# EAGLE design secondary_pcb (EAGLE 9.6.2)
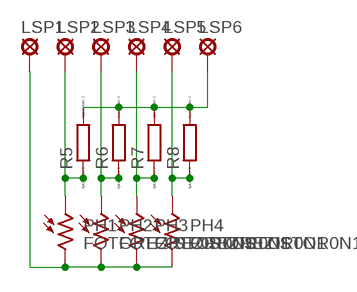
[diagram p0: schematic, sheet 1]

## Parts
LSP1  SVORKA_2,3/0,8  [LSP10]
LSP2  SVORKA_2,3/0,8  [LSP10]
LSP3  SVORKA_2,3/0,8  [LSP10]
LSP4  SVORKA_2,3/0,8  [LSP10]
LSP5  SVORKA_2,3/0,8  [LSP10]
LSP6  SVORKA_2,3/0,8  [LSP10]
PH1  FOTOREZISTOR0N1  [VT800]
PH2  FOTOREZISTOR0N1  [VT800]
PH3  FOTOREZISTOR0N1  [VT800]
PH4  FOTOREZISTOR0N1  [VT800]
R5  R0207/10  [0207/10]
R6  R0207/10  [0207/10]
R7  R0207/10  [0207/10]
R8  R0207/10  [0207/10]

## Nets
N$1: LSP1.MP PH1.2 PH2.2 PH3.2 PH4.2
N$2: LSP2.MP PH1.1 R5.1
N$3: LSP3.MP PH2.1 R6.1
N$4: LSP4.MP PH3.1 R7.1
N$5: LSP5.MP PH4.1 R8.1
N$6: LSP6.MP R5.2 R6.2 R7.2 R8.2

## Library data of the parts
LSP1-LSP6 = knihovna praxe 123:SVORKA_2,3/0,8: SOLDER PAD
PH1-PH4 = knihovna praxe 123:FOTOREZISTOR: Photoconductive Cell VT800 Series
R5-R8 = eagle-ltspice:R: RESISTOR, European symbol; SPICEMODEL: NONE; SPICEPREFIX: R

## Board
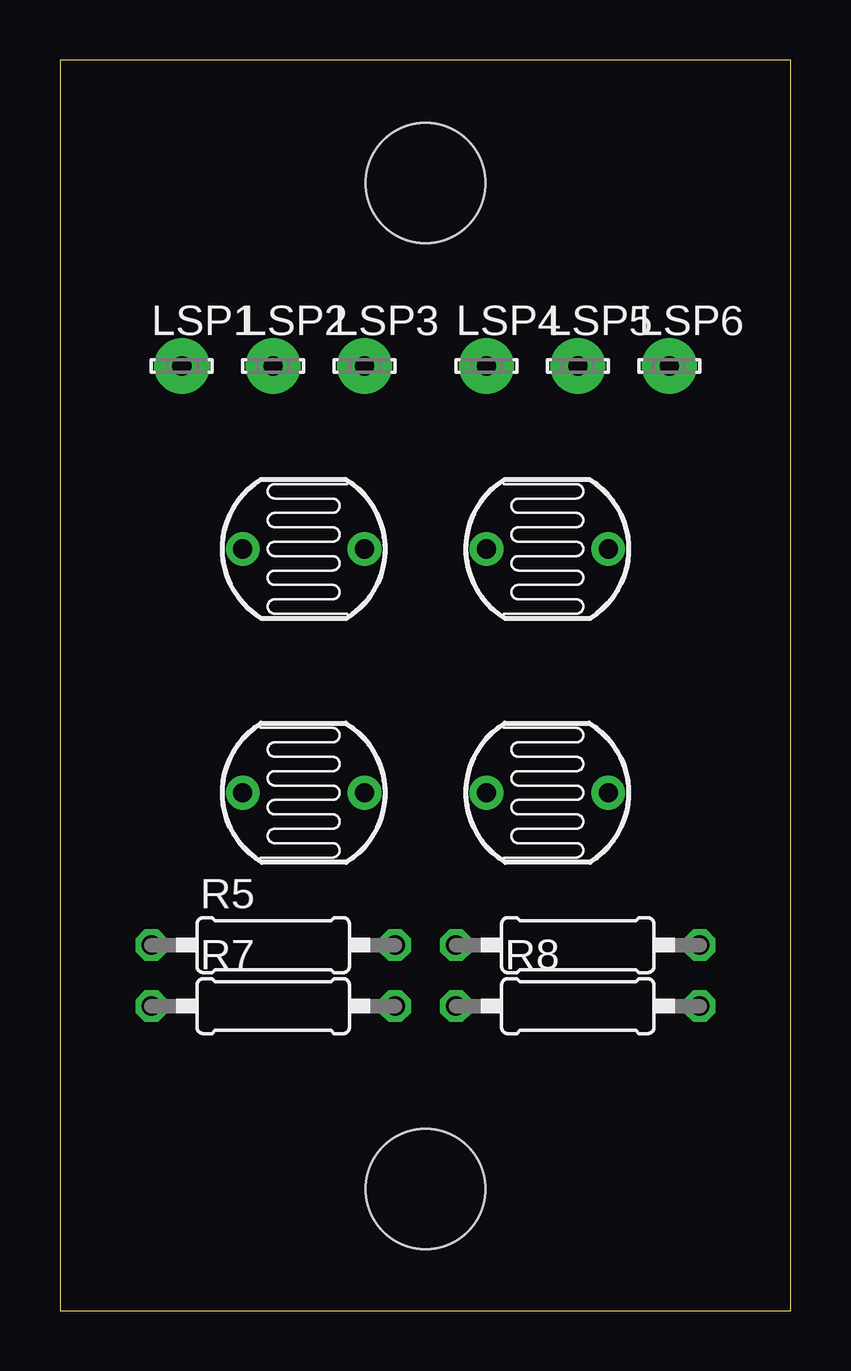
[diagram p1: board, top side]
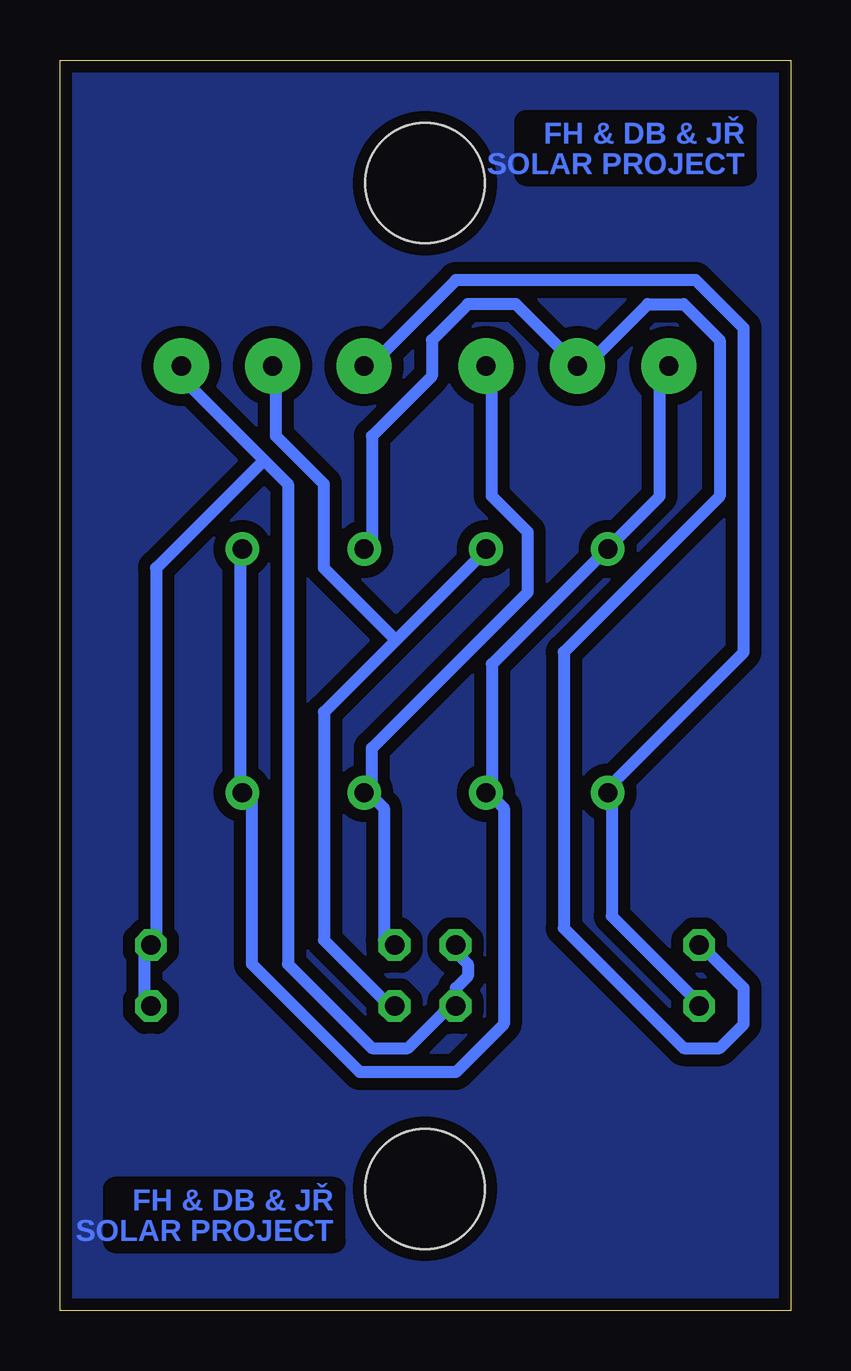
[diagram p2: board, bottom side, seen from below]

Size 30.46 x 52.12 mm. Coordinates in mm from the lower left corner, seen from the top.
Outline: 0,0 30.46,0 30.46,52.12 0,52.12 0,0
Copper layers (1*16): Top 0.035mm / dielectric 1.5mm / Bottom 0.035mm
Design rules "default *": minimum track width 0.5mm, minimum drill 1mm, track to track 0.5mm, track to pad 0.7mm, pad to pad 0.3mm, via to via 0.5mm, smd to smd 0.3mm, copper to edge 0.5mm, drill to drill 0.5mm, minimum pad ring 10mil, minimum via ring 8mil, stop-mask expansion 4mil, vias tented up to drill 0mil, thermal gap 10mil
Holes 5 mm at 15.24,5.08 15.24,46.99

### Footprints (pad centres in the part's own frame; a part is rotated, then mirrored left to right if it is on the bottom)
LSP10 = drill 0.8 pad 2.3: MP 0,0
VT800 = drill 0.8 pad 1.4: 1 -2.54,0; 2 2.54,0
0207/10 = drill 0.813 octagon: 1 -5.08,0; 2 5.08,0

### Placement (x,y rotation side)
LSP1  5.08,39.37 0 top
LSP2  8.89,39.37 0 top
LSP3  12.7,39.37 0 top
LSP4  17.78,39.37 0 top
LSP5  21.59,39.37 0 top
LSP6  25.4,39.37 0 top
PH1  20.32,31.75 0 top
PH2  20.32,21.59 0 top
PH3  10.16,21.59 0 top
PH4  10.16,31.75 180 top
R5  8.89,15.24 0 top
R6  21.59,15.24 0 top
R7  8.89,12.7 0 top
R8  21.59,12.7 0 top

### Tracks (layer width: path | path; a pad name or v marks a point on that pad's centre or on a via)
GND
  pour Bottom: 0,52.07 30.48,52.07 30.48,0 0,0
N$1
  Bottom 0.5: PH1.2 22.96,31.45 22.96,21.95 PH2.2 22.46,21.45 22.46,14.45 17.96,9.95 13.96,9.95 11.96,11.95 11.96,20.95 12.46,21.45 PH3.2 12.46,21.95 12.46,26.95 7.96,31.45 PH4.2 7.46,31.95 5.46,33.95 5.46,38.95 LSP1.MP
N$2
  Bottom 0.5: R5.1 3.46,14.95 1.96,13.45 1.96,11.95 2.96,10.95 4.46,10.95 9.46,15.95 9.46,27.45 2.96,33.95 2.96,40.45 4.46,41.95 5.96,41.95 8.46,39.45 LSP2.MP 8.96,39.45 11.46,41.95 13.46,41.95 14.96,40.45 14.96,38.95 17.46,36.45 17.46,31.95 PH1.1
N$3
  Bottom 0.5: R6.1 16.96,15.45 16.96,20.95 17.46,21.45 PH2.1 17.46,21.95 17.46,23.45 10.96,29.95 10.96,32.45 12.46,33.95 12.46,38.95 LSP3.MP
N$4
  Bottom 0.5: R7.1 3.96,12.95 7.46,16.45 7.46,21.45 PH3.1 7.46,21.95 1.96,27.45 1.96,40.95 3.96,42.95 13.96,42.95 17.46,39.45 LSP4.MP
N$5
  Bottom 0.5: 16.46,27.95 12.96,31.45 PH4.1 | 16.46,27.95 19.46,24.95 19.46,15.45 16.96,12.95 R8.1 | 16.46,27.95 19.46,30.95 19.46,34.45 21.46,36.45 21.46,38.95 LSP5.MP
N$6
  Bottom 0.5: R8.2 26.96,12.95 26.96,14.95 R6.2 26.46,15.45 26.46,30.95 21.96,35.45 | R5.2 13.96,14.95 13.46,14.45 13.46,13.95 13.96,13.45 13.96,12.95 R7.2 14.46,12.45 15.96,10.95 17.46,10.95 20.96,14.45 20.96,34.45 21.96,35.45 | 21.96,35.45 25.46,38.95 LSP6.MP

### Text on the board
Bottom: FH & DB & JŘ / SOLAR PROJECT | FH & DB & JŘ / SOLAR PROJECT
